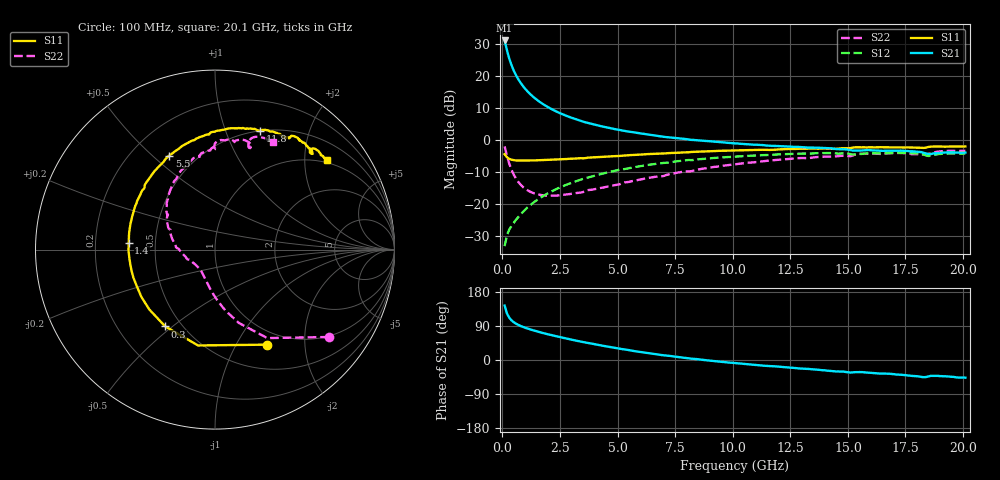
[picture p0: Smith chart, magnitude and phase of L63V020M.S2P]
!  Infineon Technologies AG
! BFR380L3 , PF131585-7, No.6, Th 09.10.01, soldered on pcb-board, measured with PP GSG850
!  Vce=3.0 V,  Ic=20.0 mA
! Common Emitter S-Parameters:  15. November 2001
#  GHz  S  MA  R  50
! f  S11  S21  S12  S22
! GHz  Mag  Ang  Mag  Ang  Mag  Ang  Mag  Ang
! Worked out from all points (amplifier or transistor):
!   201 points, 100 MHz to 20.1 GHz, reference 50 ohm
!   highest |S21| = 31.1 dB at 100 MHz (marker M1)
!   |S21| within 3 dB of that: start of sweep to 199.5 MHz
!   unconditionally stable (mu >= 1): 1.443 GHz to 4.355 GHz
!   at 3.4 GHz: K = 1.02, MAG = 8.4 dB, |S12| = -12.3 dB
!   at 10.1 GHz: K = 0.96, MSG = 2.1 dB, |S12| = -5.1 dB
!   at 20.1 GHz: K = 0.98, MSG = 0.1 dB, |S12| = -4.1 dB
!   S11 on the Smith chart (normalised r, x): 100 MHz: 0.81, -1.35; 300 MHz: 0.41, -0.47; 1.4 GHz: 0.35, +0.03; 5.5 GHz: 0.36, +0.57; 11.8 GHz: 0.50, +1.32; 20.1 GHz: 0.93, +2.54
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0.1  0.6036 -61.3  35.93 143.7  0.02214 63.3  0.7997 -37.5
0.2  0.5424 -100.0  25.4 123.0  0.03271 56.0  0.5728 -59.4
0.3  0.5101 -122.9  18.84 111.7  0.04013 54.1  0.4305 -71.9
0.4  0.4952 -137.8  14.79 104.6  0.04577 54.9  0.3438 -80.4
0.5  0.4875 -147.4  12.1 99.5  0.05148 56.6  0.2875 -86.9
0.6  0.481 -155.0  10.22 95.6  0.05761 58.1  0.2495 -92.0
0.7  0.4807 -160.9  8.839 92.5  0.06349 59.2  0.2215 -96.7
0.8  0.4796 -165.8  7.789 89.6  0.06987 60.5  0.2011 -100.7
1  0.4793 -173.4  6.291 85.0  0.08276 62.1  0.1736 -107.8
1.2  0.482 -179.6  5.279 80.9  0.0957 62.9  0.1572 -114.1
1.4  0.4826 175.5  4.554 77.3  0.1092 63.4  0.1469 -119.7
1.8  0.4888 166.8  3.582 70.6  0.1361 63.1  0.137 -129.4
2.2  0.4956 159.5  2.968 64.7  0.1628 61.8  0.1364 -138.1
2.8  0.5074 149.6  2.383 56.4  0.2025 59.1  0.1421 -149.2
3.5  0.5209 139.4  1.949 47.4  0.2484 55.2  0.1544 -159.0
5.5  0.5827 116.0  1.356 26.1  0.365 42.3  0.223 172.4
6.8  0.6174 103.0  1.156 14.0  0.4334 33.1  0.2717 156.8
10.1  0.6907 78.3  0.8894 -8.1  0.5542 11.6  0.42 125.7
11.8  0.7077 69.3  0.8136 -16.5  0.593 1.4  0.4857 111.0
13.5  0.7367 60.9  0.7645 -24.7  0.6207 -9.0  0.5358 98.8
16.8  0.7725 48.2  0.6852 -36.1  0.6276 -25.0  0.6254 77.9
20.1  0.797 38.7  0.6401 -46.6  0.6216 -38.6  0.6818 61.8
